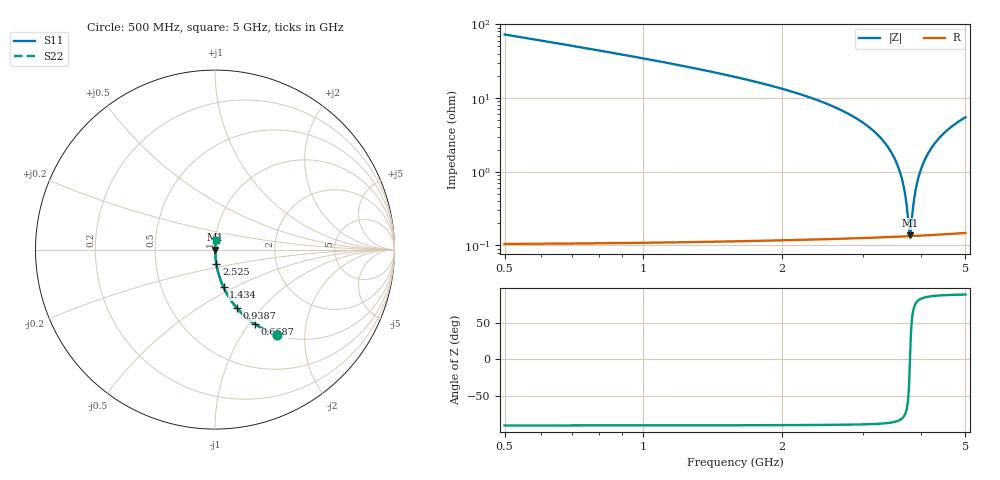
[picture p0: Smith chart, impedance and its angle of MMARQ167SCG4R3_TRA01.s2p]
! MMARQ167SCG4R3_TRA01  S-PARAMETER MODEL  ( General Type )
! Model Generated by TAIYO YUDEN Corporation (http://www.ty-top.com)
! Version 1.0
! TAIYO YUDEN Control No. 160201
! Copyright(c) 2016 TAIYO YUDEN CO.,LTD. All Rights Reserved.
! Product Description (link to TY-COMPAS)
! https://ds.yuden.co.jp/TYCOMPAS/or/detail?pn=MMARQ167SCG4R3BTRA01&u=M
! Products Name : Multilayer Ceramic Capacitors
! Characteristics :
!  Capacitance : 4.3 pF , Rated Voltage : 250V , TCC : CG / C0G
!  Case Size : 1.6 x 0.8 / 0.063 x 0.031 [mm/inch] , Thickness : 0.7 / 0.028 [mm/inch]
!  (Conditions: Temperature = 25 degC , DC Bias Current/Voltage = 0A / 0V)
! External Node Assignments :
!  1  o---| |---o  2
! GND o---------o GND
! Frequency Range : 500MHz  -  5000MHz  [ 401 STEP ]
# MHz S RI R 50
! Freq[MHz].  S11 Real  S11 Imag  S21 Real  S21 Imag  S12 Real  S12 Imag  S22 Real  S22 Imag
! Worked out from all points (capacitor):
!   401 points, 500 MHz to 5 GHz, reference 50 ohm
!   read as one part in series: C = 4.3 pF near 522.5 MHz
!   lowest |Z| = 137 mohm at 3.796 GHz (marker M1)
!   series resonance near 3.791 GHz, so ESL is about 410 pH
!   S11 on the Smith chart (normalised r, x): 500 MHz: 1.00, -1.46; 668.8 MHz: 1.00, -1.07; 938.8 MHz: 1.00, -0.74; 1.434 GHz: 1.00, -0.44; 2.525 GHz: 1.00, -0.16; 5 GHz: 1.00, +0.11
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500  0.3463 -0.4751  0.6537 0.4751  0.6537 0.4751  0.3463 -0.4751
668.75  0.2238 -0.4158  0.7762 0.4158  0.7762 0.4158  0.2238 -0.4158
938.75  0.1212 -0.3249  0.8788 0.3249  0.8788 0.3249  0.1212 -0.3249
1253.75  0.0656 -0.2454  0.9344 0.2454  0.9344 0.2454  0.0656 -0.2454
1433.75  0.0476 -0.2104  0.9524 0.2104  0.9524 0.2104  0.0476 -0.2104
2007.5  0.0184 -0.1301  0.9816 0.1301  0.9816 0.1301  0.0184 -0.1301
2525  0.0078 -0.0808  0.9922 0.0808  0.9922 0.0808  0.0078 -0.0808
2750  0.00527 -0.0633  0.9947 0.0633  0.9947 0.0633  0.00527 -0.0633
3211.25  0.00233 -0.0324  0.9977 0.0324  0.9977 0.0324  0.00233 -0.0324
3503.75  0.00154 -0.0153  0.9985 0.0153  0.9985 0.0153  0.00154 -0.0153
3593.75  0.00142 -0.0104  0.9986 0.0104  0.9986 0.0104  0.00142 -0.0104
3661.25  0.00137 -0.00678  0.9986 0.00678  0.9986 0.00678  0.00137 -0.00678
3717.5  0.00134 -0.00381  0.9987 0.00381  0.9987 0.00381  0.00134 -0.00381
3773.75  0.00134 -0.000882  0.9987 0.000882  0.9987 0.000882  0.00134 -0.000882
3796.25  0.00134 0.000275  0.9987 -0.000275  0.9987 -0.000275  0.00134 0.000275
3807.5  0.00134 0.000851  0.9987 -0.000851  0.9987 -0.000851  0.00134 0.000851
3875  0.00136 0.00427  0.9986 -0.00427  0.9986 -0.00427  0.00136 0.00427
3953.75  0.00142 0.00819  0.9986 -0.00819  0.9986 -0.00819  0.00142 0.00819
4077.5  0.00157 0.0142  0.9984 -0.0142  0.9984 -0.0142  0.00157 0.0142
4257.5  0.0019 0.0226  0.9981 -0.0226  0.9981 -0.0226  0.0019 0.0226
4572.5  0.00277 0.0367  0.9972 -0.0367  0.9972 -0.0367  0.00277 0.0367
5000  0.00445 0.0544  0.9956 -0.0544  0.9956 -0.0544  0.00445 0.0544
